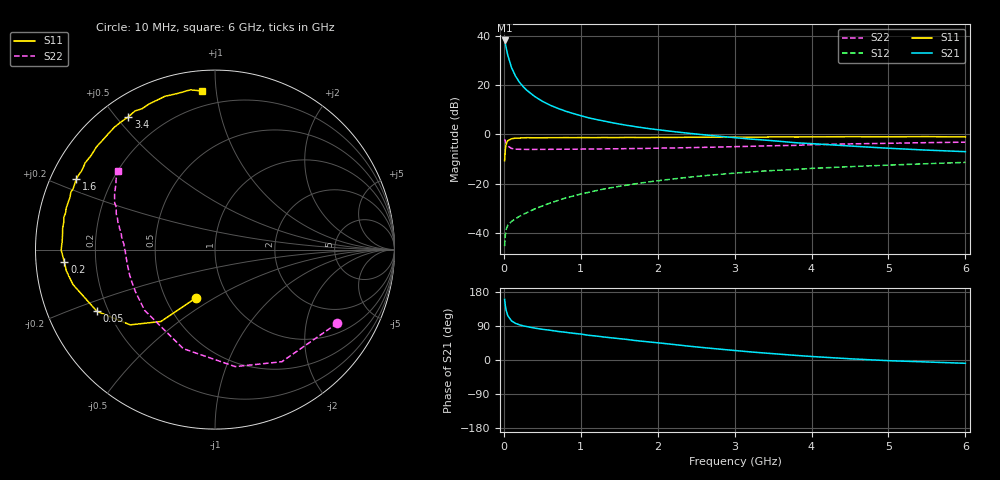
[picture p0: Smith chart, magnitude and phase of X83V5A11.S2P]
! SIEMENS Small Signal Semiconductors
! BFP136W
! Si NPN RF Bipolar Junction Transistor in SOT343
! VCE = 3.5 V  IC = 110 mA
! Common Emitter S-Parameters:  September  1994
# GHz  S  MA  R  50
!  f  S11  S21  S12  S22
! GHz  MAG  ANG  MAG  ANG  MAG  ANG  MAG  ANG
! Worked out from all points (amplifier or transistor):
!   40 points, 10 MHz to 6 GHz, reference 50 ohm
!   highest |S21| = 38.2 dB at 10 MHz (marker M1)
!   |S21| within 3 dB of that: start of sweep to 30.74 MHz
!   unconditionally stable (mu >= 1): 489.8 MHz to 2.905 GHz
!   at 200 MHz: K = 0.71, MSG = 27.4 dB, |S12| = -33.4 dB
!   at 1.5 GHz: K = 1.10, MAG = 10.8 dB, |S12| = -21.1 dB
!   at 6 GHz: K = 0.97, MSG = 2.2 dB, |S12| = -11.4 dB
!   S11 on the Smith chart (normalised r, x): 10 MHz: 0.70, -0.42; 50 MHz: 0.16, -0.24; 200 MHz: 0.09, -0.04; 1.6 GHz: 0.08, +0.24; 3.4 GHz: 0.08, +0.54; 6 GHz: 0.11, +0.92
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0.01  0.2906 -111.7  81.69 159.9  0.0053 69.5  0.7958 -31.0
0.02  0.5008 -126.9  69.69 143.2  0.0091 56.4  0.7273 -59.2
0.03  0.6316 -138.4  58.57 131.4  0.0116 49.2  0.6615 -80.2
0.05  0.7424 -152.4  41.55 117.4  0.014 40.0  0.5795 -107.8
0.1  0.8149 -166.2  22.86 103.2  0.0169 36.8  0.5179 -139.2
0.15  0.8369 -171.9  15.55 96.9  0.0191 40.4  0.5016 -152.1
0.2  0.8417 -175.2  11.67 93.1  0.0213 42.6  0.497 -159.0
0.25  0.85 -177.9  9.416 90.2  0.0236 45.9  0.4962 -163.4
0.3  0.8572 -179.8  7.873 88.1  0.0255 48.1  0.4948 -166.4
0.4  0.8527 176.8  5.929 84.2  0.0303 52.9  0.4952 -170.4
0.5  0.8538 174.1  4.73 81.1  0.0348 55.6  0.4958 -173.2
0.6  0.857 172.1  3.944 78.6  0.04 57.6  0.497 -175.0
0.7  0.8564 169.7  3.399 75.5  0.0451 59.9  0.498 -176.3
0.9  0.8572 166.1  2.663 70.6  0.0554 61.0  0.4999 -178.9
1.1  0.8594 161.8  2.176 65.3  0.0661 61.3  0.5038 179.5
1.6  0.8669 153.1  1.529 54.3  0.0927 60.0  0.5132 175.4
2.2  0.8668 142.9  1.143 41.1  0.1238 55.4  0.5285 170.8
3.2  0.883 126.0  0.804 21.5  0.1711 45.9  0.5711 162.1
3.4  0.8833 123.1  0.764 18.2  0.1806 43.7  0.584 160.3
4.5  0.8984 108.1  0.58 3.2  0.2205 33.4  0.6408 150.8
5.5  0.9006 98.8  0.478 -5.2  0.253 25.7  0.6795 144.1
6  0.8865 94.6  0.445 -8.7  0.2691 21.3  0.6945 141.2
